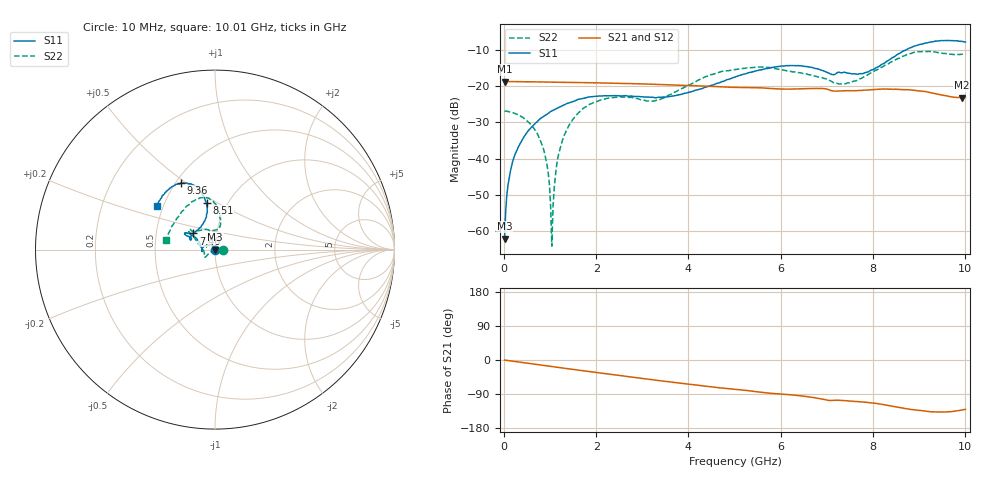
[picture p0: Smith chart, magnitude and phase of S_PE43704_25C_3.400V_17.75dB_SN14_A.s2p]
! Device ID: PE43704
! Dir: z:\PE43704\PE43704_Char_1_20130516\PE43704\AMB\3p400V\17p75dB
! Serial: 14
! Insertion: A
! Impedance: 50 ohm
! Temp: Amb
! VDD: 3.400V
! Attenuation Step: 17.75dB
! IDD: 1.138780e-01mA
#  Hz  S  RI  R  50
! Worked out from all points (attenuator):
!   401 points, 10 MHz to 10.01 GHz, reference 50 ohm
!   highest |S21| = -18.75 dB at 10 MHz (marker M1); lowest = -23.2 dB at 9.935 GHz (marker M2)
!   lowest |S11| = -62.0 dB at 10 MHz (marker M3), VSWR 1.00, Z = 50.1 + j0.0407 ohm
!   |S11| at or under -10 dB: start of sweep to 8.726 GHz
!   |S22| runs from -64.1 to -10.4 dB; largest |S21 - S12| = 0.0012
!   S11 on the Smith chart (normalised r, x): 10 MHz: 1.00, +0.00; 7.46 GHz: 0.77, +0.14; 8.51 GHz: 0.80, +0.45; 9.36 GHz: 0.53, +0.48; 10.01 GHz: 0.46, +0.27
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1e7  0.000683 0.000407  0.1155 -0.00045  0.1155 -0.000378  0.0452 -4.82e-05
1.1e8  0.000654 0.00542  0.1152 -0.00399  0.1151 -0.0039  0.0442 0.00127
2.6e8  -0.00146 0.0123  0.1146 -0.009  0.1146 -0.00896  0.0411 0.0039
5.85e8  -0.0116 0.0242  0.1128 -0.0196  0.1128 -0.0195  0.0286 0.00648
8.1e8  -0.0226 0.0287  0.1108 -0.0268  0.1109 -0.0267  0.0157 0.00426
9.1e8  -0.0277 0.029  0.1099 -0.0299  0.1099 -0.0298  0.00914 0.00265
9.85e8  -0.0317 0.0296  0.1091 -0.0322  0.1091 -0.0321  0.0041 0.00111
1.035e9  -0.0349 0.0291  0.1085 -0.0337  0.1085 -0.0336  0.000152 -0.000605
1.085e9  -0.0374 0.0286  0.108 -0.0353  0.108 -0.0352  -0.00297 -0.00234
1.16e9  -0.0416 0.0277  0.1069 -0.0375  0.1069 -0.0375  -0.00863 -0.00493
1.26e9  -0.0467 0.0262  0.1056 -0.0405  0.1056 -0.0404  -0.0154 -0.00818
1.685e9  -0.0652 0.0141  0.0988 -0.0523  0.0989 -0.0522  -0.0392 -0.0267
2.36e9  -0.0733 -0.00497  0.0855 -0.0683  0.0856 -0.0683  -0.0557 -0.0416
3.36e9  -0.0703 -0.00208  0.0613 -0.0854  0.0615 -0.0853  -0.0641 -0.006
5.01e9  -0.1128 0.07  0.021 -0.0936  0.0212 -0.0937  -0.1409 0.0929
6.685e9  -0.1618 0.0795  -0.0136 -0.0914  -0.0139 -0.0915  -0.0924 0.1058
7.46e9  -0.1207 0.0901  -0.0268 -0.0822  -0.0266 -0.0821  0.00401 0.1111
8.36e9  -0.0438 0.2256  -0.0462 -0.0778  -0.0461 -0.0784  0.0226 0.206
8.51e9  -0.047 0.2606  -0.0506 -0.0747  -0.0502 -0.0753  0.0128 0.2329
9.36e9  -0.1881 0.371  -0.0577 -0.0536  -0.0573 -0.0534  -0.1333 0.2632
9.935e9  -0.3111 0.2706  -0.0463 -0.0515  -0.0468 -0.0514  -0.2601 0.0883
1.001e10  -0.3224 0.2439  -0.0455 -0.0536  -0.0462 -0.0535  -0.271 0.0553
